{attribute 'call_after_init'}
FUNCTION_BLOCK FB_DS_IED_LD1_LLN0_DS7 EXTENDS FB_AcsiCommonDataSetClass
VAR
END_VAR

METHOD OnInit : BOOL
VAR
END_VAR
IF NOT DeleteAllMembers() THEN RETURN; END_IF
IF NOT AddMember(ipData:=fbIED.IEDLD1.CSWI1.Pos, eFc:=E_AcsiFc.ST_) THEN RETURN; END_IF
OnInit:= TRUE;
END_METHOD

END_FUNCTION_BLOCK
